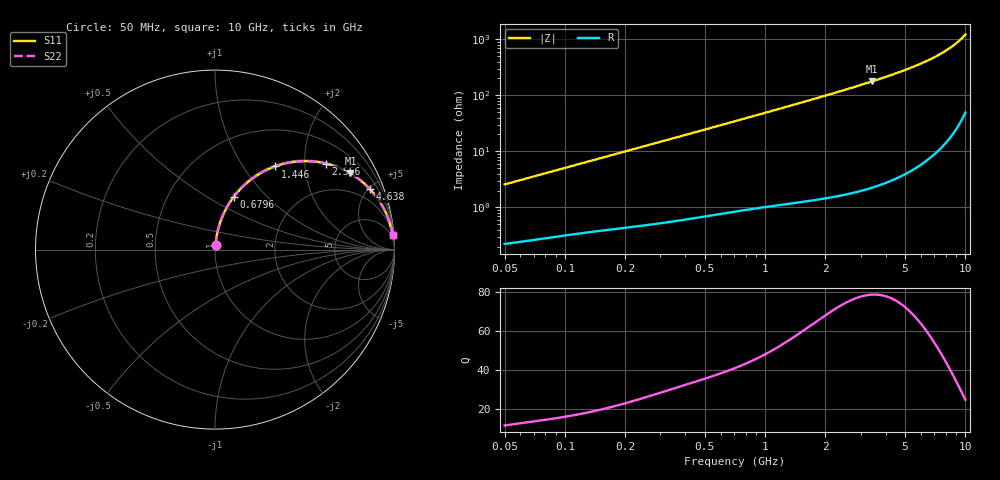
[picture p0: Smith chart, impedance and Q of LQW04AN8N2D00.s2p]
!Murata Part Number: LQW04AN8N2D00
!These Parameters are Measured in Series Mode Connection
!  o--[Z]--o
!Port1  Port2
!  o-------o
!Freq. Start=50[MHz] Stop=10[GHz], 401[Steps]
# Hz S RI R 50
!Freq.(Hz)	S 11(Real)	S 11(Imag)	S 21(Real)	S 21(Imag)	S 12(Real)	S 12(Imag)	S 22(Real)	S 22(Imag)
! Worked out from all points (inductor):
!   401 points, 50 MHz to 10 GHz, reference 50 ohm
!   read as one part in series: L = 8.1 nH near 51.34 MHz
!   highest Q = 78.6 at 3.42 GHz (marker M1), where L = 8.22 nH
!   S11 on the Smith chart (normalised r, x): 50 MHz: 1.00, +0.05; 679.6 MHz: 1.02, +0.66; 1.446 GHz: 1.02, +1.41; 2.556 GHz: 1.03, +2.56; 4.638 GHz: 1.07, +5.12; 10 GHz: 2, +24
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5e7  0.00288 0.0255  0.9971 -0.0255  0.9971 -0.0255  0.00288 0.0255
1.214486e8  0.0071 0.0601  0.9929 -0.0601  0.9929 -0.0601  0.0071 0.0601
1.956524e8  0.0134 0.0951  0.9866 -0.0951  0.9866 -0.0951  0.0134 0.0951
2.949953e8  0.0254 0.1406  0.9746 -0.1406  0.9746 -0.1406  0.0254 0.1406
4.689809e8  0.0556 0.2151  0.9444 -0.2151  0.9444 -0.2151  0.0556 0.2151
6.795592e8  0.1046 0.2939  0.8954 -0.2939  0.8954 -0.2939  0.1046 0.2939
7.071068e8  0.1119 0.3032  0.8881 -0.3032  0.8881 -0.3032  0.1119 0.3032
8.511793e8  0.1519 0.3479  0.8481 -0.3479  0.8481 -0.3479  0.1519 0.3479
1.011124e9  0.1997 0.3896  0.8003 -0.3896  0.8003 -0.3896  0.1997 0.3896
1.201124e9  0.2588 0.4286  0.7412 -0.4286  0.7412 -0.4286  0.2588 0.4286
1.445853e9  0.335 0.4634  0.665 -0.4634  0.665 -0.4634  0.335 0.4634
1.717543e9  0.4159 0.485  0.5841 -0.485  0.5841 -0.485  0.4159 0.485
2.095058e9  0.5167 0.4926  0.4833 -0.4926  0.4833 -0.4926  0.5167 0.4926
2.555552e9  0.6187 0.4791  0.3813 -0.4791  0.3813 -0.4791  0.6187 0.4791
3.420121e9  0.7545 0.4241  0.2455 -0.4241  0.2455 -0.4241  0.7545 0.4241
4.171863e9  0.8303 0.369  0.1697 -0.369  0.1697 -0.369  0.8303 0.369
4.638213e9  0.8641 0.336  0.1359 -0.336  0.1359 -0.336  0.8641 0.336
5.965537e9  0.9266 0.253  0.0734 -0.253  0.0734 -0.253  0.9266 0.253
7.37379e9  0.9619 0.1818  0.0381 -0.1818  0.0381 -0.1818  0.9619 0.1818
7.983737e9  0.9716 0.1553  0.0284 -0.1553  0.0284 -0.1553  0.9716 0.1553
8.644138e9  0.9795 0.129  0.0205 -0.129  0.0205 -0.129  0.9795 0.129
1e10  0.99 0.0812  0.00999 -0.0812  0.00999 -0.0812  0.99 0.0812
